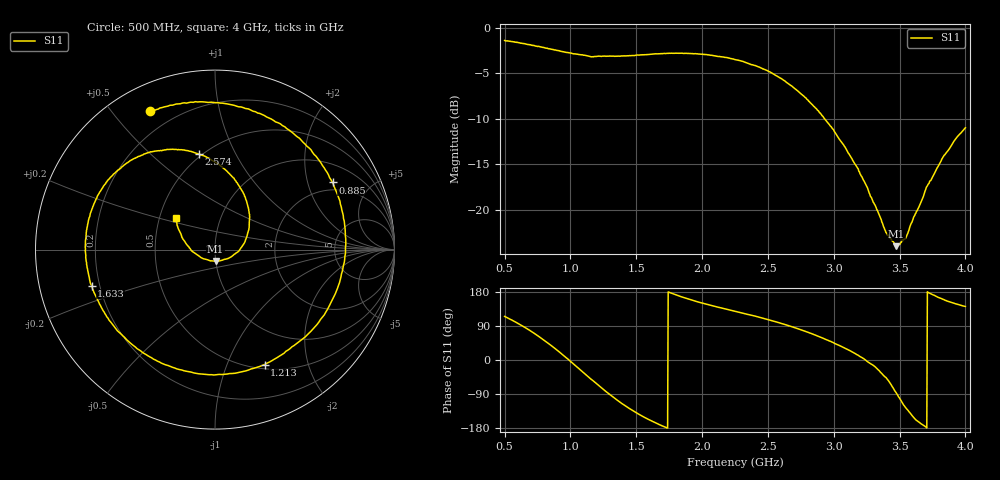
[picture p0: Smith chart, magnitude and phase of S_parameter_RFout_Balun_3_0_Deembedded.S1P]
!Agilent Technologies,E5071B,MY42403504,A.06.51
!Date: Wed Feb 26 14:55:08 2014
!Data & Calibration Information:
!Freq	S11:SOLT1(ON)
# Hz S dB R 50
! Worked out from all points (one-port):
!   801 points, 500 MHz to 4 GHz, reference 50 ohm
!   lowest |S11| = -24.0 dB at 3.475 GHz (marker M1), VSWR 1.13, Z = 49.9 - j6.3 ohm
!   |S11| at or under -10 dB: 2.929 GHz to end of sweep
!   S11 on the Smith chart (normalised r, x): 500 MHz: 0.11, +0.63; 885 MHz: 1.66, +2.89; 1.213 GHz: 0.55, -1.37; 1.633 GHz: 0.17, -0.14; 2.574 GHz: 0.48, +0.73; 4 GHz: 0.61, +0.23
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5e8  -1.41 115.0
6.00625e8  -1.64 96.7
7.0125e8  -1.90 75.8
7.93125e8  -2.18 53.9
8.85e8  -2.45 29.7
9.375e8  -2.62 14.9
9.9875e8  -2.80 -2.9
1.064375e9  -2.96 -22.6
1.134375e9  -3.11 -44.2
1.213125e9  -3.13 -66.7
1.291875e9  -3.14 -89.1
1.375e9  -3.14 -110.9
1.501875e9  -3.03 -139.4
1.633125e9  -2.90 -163.8
1.8125e9  -2.81 170.4
2.0225e9  -2.96 148.0
2.25e9  -3.51 128.5
2.420625e9  -4.27 114.3
2.57375e9  -5.37 99.4
2.6875e9  -6.49 87.0
2.90625e9  -9.55 59.3
3.125e9  -14.10 24.3
3.39625e9  -22.52 -46.0
3.475e9  -24.02 -86.9
3.5625e9  -22.62 -132.5
3.71125e9  -17.39 179.9
3.820625e9  -14.46 161.6
4e9  -11.01 141.3
